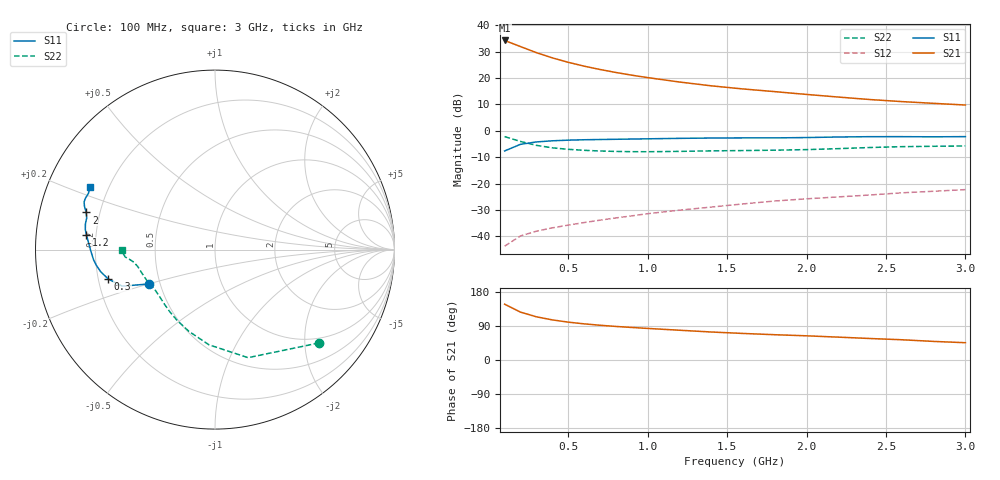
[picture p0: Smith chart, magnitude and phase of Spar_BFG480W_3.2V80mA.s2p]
! Filename: 3_280BFG480.001
! Title: BFG480W
! Bias: Vce=3.2V; Ic=80mA
! Company: NXP Semiconductors NL
! User: Quality&Reliability T&D
! Measure time: 10 Nov 1999 / 11:57:34
#  MHz  S  MA  R 50
! Freq  S11  S21  S12  S22  :
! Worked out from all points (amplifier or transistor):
!   20 points, 100 MHz to 3 GHz, reference 50 ohm
!   highest |S21| = 34.2 dB at 100 MHz (marker M1)
!   |S21| within 3 dB of that: start of sweep to 229.6 MHz
!   unconditionally stable (mu >= 1): 780.6 MHz to end of sweep
!   at 400 MHz: K = 0.77, MSG = 32.2 dB, |S12| = -36.7 dB
!   at 1.2 GHz: K = 1.07, MAG = 22.7 dB, |S12| = -30.0 dB
!   at 3 GHz: K = 1.05, MAG = 14.6 dB, |S12| = -22.3 dB
!   S11 on the Smith chart (normalised r, x): 100 MHz: 0.43, -0.20; 300 MHz: 0.24, -0.13; 1.2 GHz: 0.16, +0.06; 2 GHz: 0.15, +0.14; 3 GHz: 0.13, +0.23
100  0.4164 -152.6  51.56 147.3  0.006546 69.2  0.779 -41.9
200  0.5556 -158.5  39.46 126.3  0.01023 59.8  0.6297 -73.0
300  0.6171 -164.6  30.31 114.0  0.01257 58.1  0.5316 -93.6
400  0.6483 -169.0  24.13 105.8  0.01455 59.2  0.4775 -107.9
500  0.6665 -172.4  19.91 99.9  0.01638 61.3  0.4469 -118.3
600  0.6786 -175.1  16.82 95.4  0.01832 63.0  0.4281 -126.1
700  0.6858 -177.5  14.55 91.7  0.02034 65.0  0.4157 -132.2
800  0.6926 -179.6  12.76 88.6  0.02243 66.7  0.4078 -137.2
900  0.6996 178.4  11.34 85.9  0.02453 68.9  0.4034 -141.5
1000  0.7069 176.6  10.2 83.3  0.02698 69.8  0.4025 -145.4
1200  0.7211 173.5  8.422 78.6  0.03146 71.6  0.4085 -151.6
1400  0.7312 171.2  7.129 73.9  0.03601 72.8  0.4178 -156.3
1600  0.7361 168.8  6.221 70.1  0.04129 73.7  0.4236 -159.8
1800  0.7362 166.2  5.533 66.7  0.04691 74.3  0.4305 -163.5
2000  0.7467 163.9  4.898 63.8  0.05164 75.0  0.4414 -167.9
2200  0.7655 161.7  4.37 60.3  0.05611 75.0  0.4604 -171.5
2400  0.7763 160.0  3.917 56.7  0.06103 74.6  0.4838 -173.9
2600  0.7765 158.3  3.583 53.4  0.06706 73.9  0.5019 -175.3
2800  0.7716 156.1  3.321 49.0  0.07178 72.5  0.5103 -177.2
3000  0.7775 153.4  3.084 45.6  0.07713 71.9  0.5176 180.0
